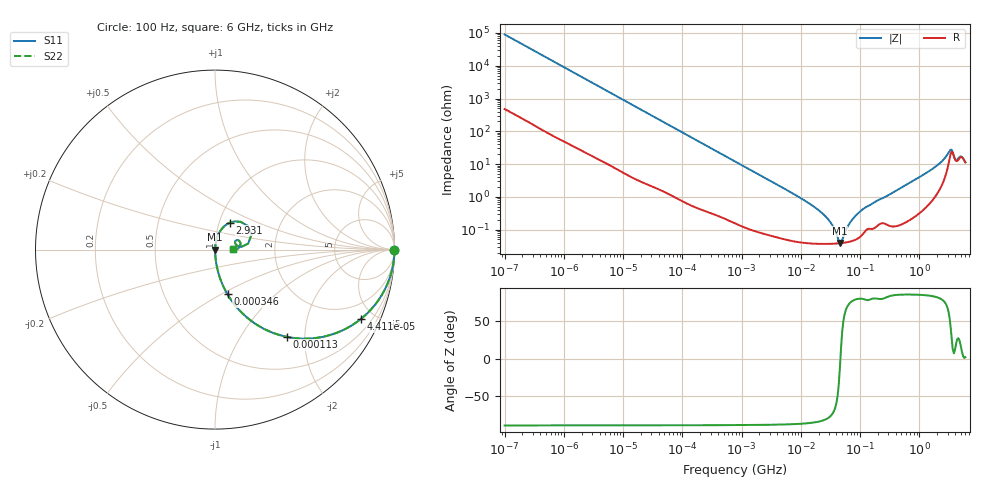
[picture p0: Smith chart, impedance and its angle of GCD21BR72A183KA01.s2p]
!Murata Part Number: GCD21BR72A183KA01
!These Parameters are Measured in Series Mode Connection
!Data Generated on Jan 08, 2026
!  o--ll--o
!Port1  Port2
!  o------o
!Operation Temp=25[degC], DC Bias Voltage=0[V]
!Freq. Start=100[Hz] Stop=6[GHz] 401[Steps]
# Hz S RI R 50
!Freq.(Hz) S11(Real) S11(Imag) S21(Real) S21(Imag) S12(Real) S12(Imag) S22(Real) S22(Imag)
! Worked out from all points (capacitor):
!   401 points, 100 Hz to 6 GHz, reference 50 ohm
!   read as one part in series: C = 17.6 nF near 109 Hz
!   lowest |Z| = 39.4 mohm at 45.56 MHz (marker M1)
!   series resonance near 46.64 MHz, so ESL is about 660 pH
!   S11 on the Smith chart (normalised r, x): 100 Hz: open; 44.11 kHz: 1.03, -4.18; 113 kHz: 1.01, -1.64; 346 kHz: 1.01, -0.54; 2.931 GHz: 1.13, +0.35; 6 GHz: 1.22, +0.01
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100  1 -0.00111  7.1e-06 0.00111  7.1e-06 0.00111  1 -0.00111
2008  0.9994 -0.022  0.00061 0.022  0.00061 0.022  0.9994 -0.022
11009  0.9851 -0.1182  0.0149 0.1182  0.0149 0.1182  0.9851 -0.1182
40335  0.8373 -0.3654  0.1627 0.3654  0.1627 0.3654  0.8373 -0.3654
44113  0.8118 -0.3872  0.1882 0.3872  0.1882 0.3872  0.8118 -0.3872
112960  0.4026 -0.4864  0.5974 0.4864  0.5974 0.4864  0.4026 -0.4864
193316  0.1894 -0.3874  0.8106 0.3874  0.8106 0.3874  0.1894 -0.3874
345986  0.0698 -0.2495  0.9302 0.2495  0.9302 0.2495  0.0698 -0.2495
774597  0.0159 -0.1188  0.9841 0.1188  0.9841 0.1188  0.0159 -0.1188
1.555665e7  0.000404 -0.00545  0.9996 0.00545  0.9996 0.00545  0.000404 -0.00545
2.911731e7  0.00037 -0.002  0.9996 0.002  0.9996 0.002  0.00037 -0.002
4.556224e7  0.000382 -9.53e-05  0.9996 9.53e-05  0.9996 9.53e-05  0.000382 -9.53e-05
4.983056e7  0.000389 0.000273  0.9996 -0.000273  0.9996 -0.000273  0.000389 0.000273
6.817316e7  0.000434 0.00161  0.9996 -0.00161  0.9996 -0.00161  0.000434 0.00161
9.326766e7  0.000554 0.00312  0.9994 -0.00312  0.9994 -0.00312  0.000554 0.00312
3.124326e8  0.00144 0.0116  0.9986 -0.0116  0.9986 -0.0116  0.00144 0.0116
1.565993e9  0.011 0.0645  0.989 -0.0645  0.989 -0.0645  0.011 0.0645
2.931063e9  0.0844 0.1508  0.9156 -0.1508  0.9156 -0.1508  0.0844 0.1508
3.352442e9  0.1817 0.1323  0.8183 -0.1323  0.8183 -0.1323  0.1817 0.1323
4.193612e9  0.1112 0.0366  0.8888 -0.0366  0.8888 -0.0366  0.1112 0.0366
5.016141e9  0.1425 0.0367  0.8575 -0.0367  0.8575 -0.0367  0.1425 0.0367
6e9  0.1011 0.00284  0.8989 -0.00284  0.8989 -0.00284  0.1011 0.00284
